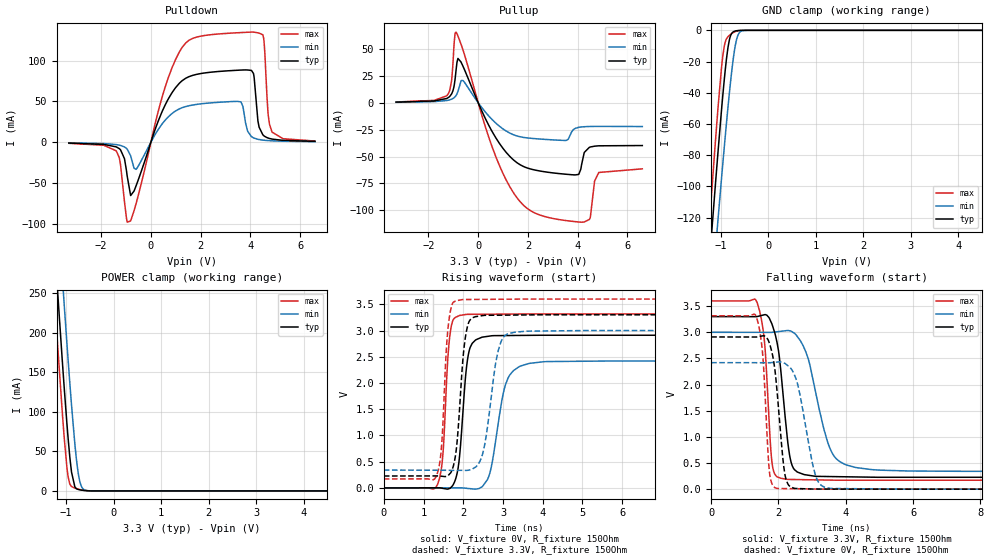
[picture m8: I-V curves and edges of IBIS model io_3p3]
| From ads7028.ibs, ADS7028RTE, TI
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|   io_3p3 Model
[Model]   io_3p3
Model_type   I/O
Polarity   Non-Inverting
Enable   Active-Low
Vinl = 0.99
Vinh = 2.31
Vmeas = 1.65
Vref = 0
Cref = 2pF
Rref = 100000
|   typ   min   max
C_comp   1.207pF   1.185pF   1.229pF
[Model spec]
|subparameter
Vinl   0.99   0.9   1.08
Vinh   2.31   2.1   2.52
| Where Nom  PVT is Nominal Process, 3.3V, 27C
|   Fast PVT is Strong Process,  3.6V, -40C
|   Slow PVT is Weak Process,   3.0V, 125C
[Voltage Range]   3.3   3   3.6
|Junction Temperature
[Temperature Range]   27   125   -40
[Pullup Reference]   3.3   3   3.6
[Pulldown Reference]   0   0   0
[Power Clamp Reference]   3.3   3   3.6
[GND Clamp Reference]   0   0   0
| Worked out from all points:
|   slope of the pulldown table from 0 to 0.495 V, typ, clamps not added: 12.2 ohm
|   slope of the pullup table from 0 to 0.495 V, typ, clamps not added: 20.6 ohm
|   GND clamp passes 1 mA (typ) near -0.73 V on its own axis
|   POWER clamp passes 1 mA (typ) near -0.67 V on its own axis
|   falling waveform, V_fixture 3.3V, R_fixture 150Ohm: 20-80 % time 297ps typ, 582ps min, 193ps max; typ from 3.3 V to 0.227 V
|   rising waveform, V_fixture 0V, R_fixture 150Ohm: 20-80 % time 183ps typ, 324ps min, 140ps max; typ from 0 V to 2.91 V
|   rising waveform, V_fixture 3.3V, R_fixture 150Ohm: 20-80 % time 182ps typ, 288ps min, 141ps max; typ from 0.227 V to 3.3 V
|   falling waveform, V_fixture 0V, R_fixture 150Ohm: 20-80 % time 247ps typ, 418ps min, 172ps max; typ from 2.91 V to 0 V
[Pulldown]
|   Voltage   I(typ)   I(min)   I(max)
-3.3V     -1.069mA   -742.8uA   -1.333mA
-1.399V   -5.682mA   -2.899mA   -10.49mA
-953.7mV  -41.5mA    -8.441mA   -98.16mA
-815.1mV  -65.44mA   -16.69mA   -96.61mA
-597.3mV  -53.65mA   -33.31mA   -75.52mA
1.244V    75.15mA    42.19mA    115.7mA
3.61V     88.51mA    49.54mA    134.5mA
4.046V    88.08mA    6.885mA    135.2mA
4.531V    8.245mA    2.488mA    128.3mA
4.719V    5.08mA     1.979mA    33.23mA
4.877V    3.818mA    1.687mA    12.35mA
6.6V      1.01mA     640.4uA    1.438mA
[GND Clamp]
|   Voltage   I(typ)   I(min)   I(max)
-3.3V     -1.016A    -995.9mA   -1.06A
-1.32V    -182.2mA   -219.5mA   -160.2mA
-1.211V   -138.4mA   -178.5mA   -113.2mA
-1.191V   -130.5mA   -171.1mA   -104.8mA
-1.063V   -80.55mA   -123.8mA   -52.33mA
-953.7mV  -41.34mA   -85.1mA    -16.15mA
-844.8mV  -10.76mA   -48.93mA   -4.045mA
-795.3mV  -3.773mA   -34.03mA   -2.68mA
-716.1mV  -691.3uA   -14.24mA   -1.157mA
-627mV    -129.5uA   -2.529mA   -272uA
-478.5mV  -4.946uA   -45.37uA   -7.702uA
6.6V      0A         0A         0A
[Pullup]
|   Voltage   I(typ)   I(min)   I(max)
-3.3V     601.2uA    425.4uA    730.1uA
-1.251V   4.184mA    2.18mA     6.912mA
-1.073V   8.15mA     3.344mA    20.29mA
-894.3mV  29.61mA    6.656mA    65.79mA
-617.1mV  34.23mA    20.72mA    49.51mA
709.5mV   -32.66mA   -18.97mA   -50.22mA
1.957V    -60.57mA   -32.66mA   -98.08mA
4.036V    -66.7mA    -22.87mA   -110.9mA
4.264V    -46.29mA   -22.28mA   -110.9mA
4.501V    -41.2mA    -22.06mA   -107.2mA
4.848V    -40.05mA   -21.96mA   -64.87mA
6.6V      -39.8mA    -22.11mA   -61.49mA
[POWER Clamp]
|   Voltage   I(typ)   I(min)   I(max)
-3.3V     2.318A     2.417A     2.257A
-1.261V   328.9mA    436.8mA    261.3mA
-1.221V   292.4mA    400.2mA    224.8mA
-1.181V   256.2mA    363.9mA    188.8mA
-1.043V   134.6mA    239.7mA    71.11mA
-953.7mV  65.06mA    163.8mA    17.31mA
-884.4mV  23.9mA     108.7mA    5.58mA
-815.1mV  5.403mA    60.07mA    3.59mA
-755.7mV  2.139mA    27.81mA    2.523mA
-706.2mV  1.338mA    11.19mA    1.769mA
-557.7mV  259.1uA    454.8uA    307.4uA
6.6V      0A         0A         0A
[Ramp]
R_load = 150
|   typ   min   max
dV/dt_r   1.74636/1.82756e-10   1.45146/3.23545e-10   1.98954/1.39929e-10
dV/dt_f   1.84365/2.9629e-10   1.5954/5.81906e-10   2.05717/1.92813e-10
[Falling Waveform]
V_fixture = 3.3V
V_fixture_min = 3V
V_fixture_max = 3.6V
R_fixture = 150Ohm
C_fixture = 0F
|   Time   V(typ)   V(min)   V(max)
0s        3.3V       3V         3.6V
1.36ns    3.3V       2.999V     3.577V
1.586ns   3.336V     2.999V     2.809V
1.831ns   3.11V      3V         411.9mV
2.013ns   2.596V     3.014V     222.7mV
2.235ns   1.156V     3.031V     189.4mV
2.473ns   374.6mV    2.982V     184.4mV
3.599ns   240.5mV    687.1mV    172.4mV
4.754ns   229.3mV    375.2mV    171.6mV
50ns      227.2mV    341mV      171.4mV
[Rising Waveform]
V_fixture = 0V
V_fixture_min = 0V
V_fixture_max = 0V
R_fixture = 150Ohm
C_fixture = 0F
|   Time   V(typ)   V(min)   V(max)
0s        -59.87nV   -61.47nV   -14.2nV
1.342ns   1.876mV    1.318mV    51.63mV
1.485ns   -8.227mV   1.459mV    620.3mV
1.69ns    10.37mV    1.66mV     3.05V
1.89ns    489.7mV    1.857mV    3.281V
2.065ns   2.177V     -5.878mV   3.307V
2.645ns   2.892V     224.8mV    3.311V
3.17ns    2.905V     2.152V     3.314V
4.024ns   2.91V      2.405V     3.316V
50ns      2.911V     2.419V     3.316V
[Rising Waveform]
V_fixture = 3.3V
V_fixture_min = 3V
V_fixture_max = 3.6V
R_fixture = 150Ohm
C_fixture = 0F
|   Time   V(typ)   V(min)   V(max)
0s        227.2mV    341mV      171.4mV
1.322ns   228.9mV    337mV      221.5mV
1.456ns   223.3mV    336.6mV    824.1mV
1.651ns   261.7mV    336mV      3.259V
1.83ns    771.5mV    335.5mV    3.569V
1.976ns   2.316V     335mV      3.59V
2.48ns    3.284V     627.4mV    3.594V
2.97ns    3.293V     2.819V     3.597V
3.545ns   3.297V     2.986V     3.6V
50ns      3.3V       3V         3.6V
[Falling Waveform]
|Gnd
V_fixture = 0V
V_fixture_min = 0V
V_fixture_max = 0V
R_fixture = 150Ohm
C_fixture = 0F
|   Time   V(typ)   V(min)   V(max)
0s        2.911V     2.419V     3.316V
1.342ns   2.909V     2.418V     3.298V
1.534ns   2.932V     2.418V     2.555V
1.734ns   2.784V     2.418V     318.1mV
1.956ns   1.891V     2.43V      14.52mV
2.281ns   97.44mV    2.36V      10.5mV
2.576ns   11.9mV     1.99V      7.713mV
3.096ns   2.613mV    273.4mV    2.797mV
3.545ns   1.661mV    14.77mV    207uV
50ns      -50.08nV   -49.31nV   1.128nV
